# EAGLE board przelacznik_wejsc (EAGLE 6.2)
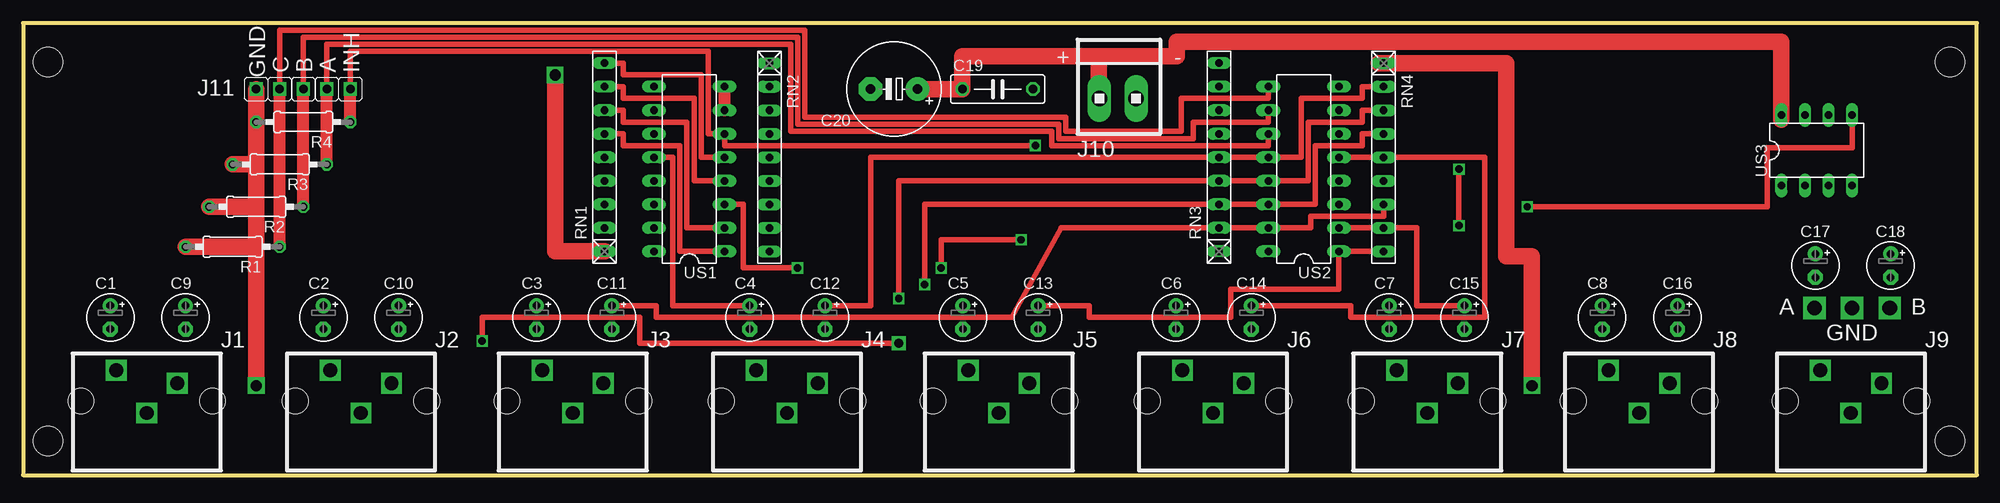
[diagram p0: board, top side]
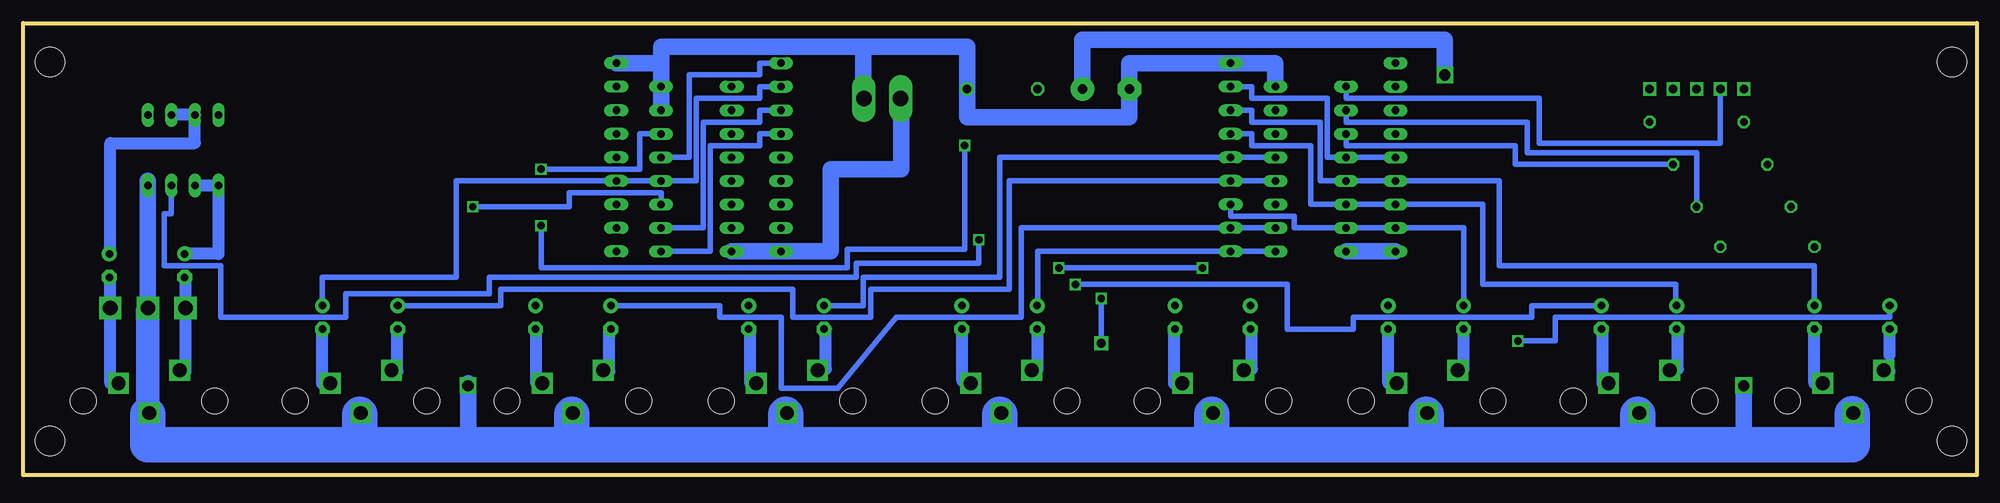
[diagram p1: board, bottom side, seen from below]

Size 210.82 x 48.77 mm. Coordinates in mm from the lower left corner, seen from the top.
Outline: 0,0 210.82,0 210.82,48.77 0,48.77 0,0
Copper layers (1*16): Top 0.035mm / dielectric 1.5mm / Bottom 0.035mm
Design rules: minimum track width 10mil, minimum drill 24mil, track to track 8mil, track to pad 8mil, pad to pad 8mil, via to via 8mil, smd to smd 8mil, copper to edge 40mil, drill to drill 8mil, minimum pad ring 10mil, minimum via ring 8mil, stop-mask expansion 4mil, vias tented up to drill 0mil, thermal gap 10mil
Holes 2.8 mm at 6.23,8 20.43,8 29.35,8 43.55,8 52.21,8 66.41,8 75.32,8 89.52,8 98.18,8 112.38,8 121.3,8 135.5,8 144.41,8 158.61,8 167.27,8 181.47,8 190.13,8 204.33,8
Holes 3.2 mm at 2.68,3.68 207.91,3.68 207.91,44.58 2.68,44.58

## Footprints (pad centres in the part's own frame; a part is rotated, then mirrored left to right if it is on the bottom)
E2,5-5 = drill 0.813 pad 1.6: + -1.27,0 | drill 0.813 pad 1.6 octagon: - 1.27,0
C075-032X103 = drill 0.914 octagon: 1 -3.81,0; 2 3.81,0
E5-10,5 = drill 1.016 pad 2.54: + -2.54,0 | drill 1.016 pad 2.54 octagon: - 2.54,0
JP1 = drill 0.914 pad 1.422 square: 1 0,-1.27; 2 0,1.27
1X2MTA = drill 1.676 long: 1 1.981,0; 2 -1.981,0
0207/10 = drill 0.813 octagon: 1 -5.08,0; 2 5.08,0
RN-9 = drill 0.813 long: 1 -10.16,0; 2 -7.62,0; 3 -5.08,0; 4 -2.54,0; 5 0,0; 6 2.54,0; 7 5.08,0; 8 7.62,0; 9 10.16,0
DIL16 = drill 0.813 long: 1 -8.89,-3.81; 2 -6.35,-3.81; 3 -3.81,-3.81; 4 -1.27,-3.81; 5 1.27,-3.81; 6 3.81,-3.81; 7 6.35,-3.81; 8 8.89,-3.81; 9 8.89,3.81; 10 6.35,3.81; 11 3.81,3.81; 12 1.27,3.81; 13 -1.27,3.81; 14 -3.81,3.81; 15 -6.35,3.81; 16 -8.89,3.81
DIL08 = drill 0.813 long: 1 -3.81,-3.81; 2 -1.27,-3.81; 3 1.27,-3.81; 4 3.81,-3.81; 5 3.81,3.81; 6 1.27,3.81; 7 -1.27,3.81; 8 -3.81,3.81

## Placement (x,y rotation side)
C1  [E2,5-5]  9.4,17.02 270 top
C2  [E2,5-5]  32.4,17.02 270 top
C3  [E2,5-5]  55.4,17.02 270 top
C4  [E2,5-5]  78.4,17.02 270 top
C5  [E2,5-5]  101.4,17.02 270 top
C6  [E2,5-5]  124.4,17.02 270 top
C7  [E2,5-5]  147.4,17.02 270 top
C8  [E2,5-5]  170.4,17.02 270 top
C9  [E2,5-5]  17.53,17.02 270 top
C10  [E2,5-5]  40.53,17.02 270 top
C11  [E2,5-5]  63.53,17.02 270 top
C12  [E2,5-5]  86.53,17.02 270 top
C13  [E2,5-5]  109.53,17.02 270 top
C14  [E2,5-5]  132.53,17.02 270 top
C15  [E2,5-5]  155.53,17.02 270 top
C16  [E2,5-5]  178.53,17.02 270 top
C17  [E2,5-5]  193.4,22.61 270 top
C18  [E2,5-5]  201.53,22.61 270 top
C19  [C075-032X103]  105.16,41.66 0 top
C20  [E5-10,5]  93.98,41.66 180 top
E$9  [JP1]  31.5,41.66 90 top
E$10  [JP1]  28.96,41.66 90 top
E$11  [JP1]  26.42,41.66 90 top
J10  [1X2MTA]  118.11,40.64 0 top
J11  [JP1]  34.04,41.66 90 top
R1  [0207/10]  22.61,24.64 180 top
R2  [0207/10]  25.15,28.96 180 top
R3  [0207/10]  27.69,33.53 180 top
R4  [0207/10]  30.23,38.1 180 top
RN1  [RN-9]  62.74,34.29 90 top
RN2  [RN-9]  80.52,34.29 270 top
RN3  [RN-9]  129.03,34.29 90 top
RN4  [RN-9]  146.81,34.29 270 top
US1  [DIL16]  71.88,33.02 90 top
US2  [DIL16]  138.18,33.02 90 top
US3  [DIL08]  193.55,35.05 0 top

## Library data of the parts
C1-C20 R1-R4 = rcl
E$9-E$11 J11 = hybrid
J10 = con-amp
RN1-RN4 = resistor-net
US1-US3 = 40xx

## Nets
S$9: C9.+ RN2.3 US1.13
S$15: E$11.2 R3.2
S$39: US2.3 US3.5
S$87: RN1.1
S$88: C19.2 C20.- RN2.1 RN4.1 US2.7 US2.8
S$89: C1.+ RN4.3 US2.13
S$90: RN2.4 US1.14
S$91: RN2.7 US1.15
S$92: RN1.5 RN2.2 US1.12
S$93: RN1.6 US1.1
S$94: RN3.1
S$95: RN1.9 US1.5
S$97: RN1.8
S$98: US1.7 US1.8
S$99: US1.4
S$100: US1.2
S$101: RN3.8 US2.4
S$102: RN3.7 US2.2
S$103: RN3.9 US2.5
S$104: RN3.6 RN4.9 US2.1
S$106: RN4.7 US2.15
S$107: US3.4
S$109: US3.6 US3.7
S$111: RN4.2 US2.12
S$113: RN4.4 US2.14
S$116: US1.3 US3.3
S$117: R2.2
S$119: R1.2
S$120: J11.2 R3.1 US1.11 US2.11
S$121: E$9.2 R2.1 US1.10 US2.10
S$123: E$10.2 R1.1 US1.9 US2.9
S$124: R4.1 US1.6 US2.6
S$128: C19.1 C20.+

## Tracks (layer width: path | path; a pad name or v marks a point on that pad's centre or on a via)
S$1  (via drill 1.5)
  other vias: 13.33,6.7
S$2  (via drill 1.5)
  other vias: 16.63,9.9
S$3  (via drill 1.5)
  other vias: 10.03,11.3
S$4  (via drill 1.5)
  other vias: 36.45,6.7
S$5  (via drill 1.5)
  other vias: 39.75,9.9
S$6  (via drill 1.5)
  other vias: 33.15,11.3
S$7
  Bottom 1.27: 33.02,11.43 32.26,11.43 32.26,15.75
S$8
  Bottom 1.27: 39.88,9.91 40.39,9.91 40.39,15.75
S$9
  Bottom 0.61: RN2.3 78.23,39.37 78.23,38.1 70.87,38.1 70.87,31.75 US1.13 51.56,31.75 51.56,22.61 17.53,22.61 C9.+
S$10  (via drill 1.5)
  other vias: 59.31,6.7
S$11  (via drill 1.5)
  other vias: 62.61,9.9
S$12  (via drill 1.5)
  other vias: 56.01,11.3
S$13
  Bottom 1.27: 56.13,11.43 55.37,11.43 55.37,15.75
S$14
  Bottom 1.27: 62.74,9.91 63.5,9.91 63.5,15.75
S$15  (via drill 1.2)
  Top 1.778: 25.15,33.53 E$11.2 | 25.15,33.53 R3.2 | v25.15,9.65 25.15,33.53
  Bottom 1.778: 25.15,5.08 v25.15,9.65
S$16  (via drill 1.5)
  other vias: 82.42,6.7
S$17  (via drill 1.5)
  other vias: 85.72,9.9
S$18  (via drill 1.5)
  other vias: 79.12,11.3
S$19
  Bottom 1.27: 102.11,11.43 101.35,11.43 101.35,15.75
S$20
  Bottom 1.27: 108.46,10.16 109.47,10.16 109.47,15.75
S$21
  Bottom 1.27: 78.99,11.43 78.23,11.43 78.23,15.75
S$22
  Bottom 3.81: 82.55,3.56 82.55,6.56
S$23  (via drill 1.5)
  other vias: 105.28,6.7
S$24  (via drill 1.5)
  other vias: 108.58,9.9
S$25  (via drill 1.5)
  other vias: 101.98,11.3
S$26
  Bottom 1.27: 85.85,9.91 86.61,9.91 86.61,15.75
S$27
  Bottom 1.27: 9.42,12.95 9.42,15.75
S$28  (via drill 1.5)
  other vias: 128.4,6.7
S$29  (via drill 1.5)
  other vias: 131.7,9.9
S$30  (via drill 1.5)
  other vias: 125.1,11.3
S$31
  Bottom 1.27: 124.97,11.43 124.21,11.43 124.21,15.75
S$32
  Bottom 1.27: 131.83,9.91 132.33,9.91 132.33,15.75
S$33  (via drill 1.2)
  Top 1.778: 146.3,44.45 160.02,44.45 160.02,23.62 162.81,23.62 v162.81,9.65
S$34  (via drill 1.5)
  other vias: 151.51,6.7
S$35  (via drill 1.5)
  other vias: 154.81,9.9
S$36  (via drill 1.5)
  other vias: 148.21,11.3
S$37
  Bottom 1.27: 148.34,11.18 147.57,11.18 147.57,15.75
S$38
  Bottom 1.27: 154.94,9.91 155.45,9.91 155.45,15.75
S$39  (via drill 0.8)
  Top 0.61: US3.5 197.36,35.31 188.21,35.31 188.21,28.96 v162.31,28.96
  Bottom 0.61: US2.3 141.99,30.48 151.89,30.48 151.89,28.96 v162.31,28.96
S$40  (via drill 1.5)
  other vias: 174.37,6.7
S$41  (via drill 1.5)
  other vias: 177.67,9.9
S$42  (via drill 1.5)
  other vias: 171.07,11.3
S$43
  Bottom 1.27: 170.43,15.75 170.43,11.18 170.94,11.18
S$45
  Bottom 3.81: 105.41,3.56 105.41,6.56
S$46
  Bottom 3.81: 128.52,3.56 128.52,6.56
S$47
  Bottom 3.81: 151.64,3.56 151.64,6.56
S$48
  Bottom 3.81: 36.58,3.56 36.58,6.56
S$49
  Bottom 3.81: 59.44,3.56 59.44,6.56
S$50
  Bottom 1.27: 177.8,9.91 178.56,9.91 178.56,15.75
S$52
  Bottom 3.81: 174.5,3.56 174.5,6.56
S$53  (via drill 1.5)
  other vias: 197.23,6.7
S$54  (via drill 1.5)
  other vias: 200.53,9.9
S$55  (via drill 1.5)
  other vias: 193.93,11.3
S$56
  Bottom 1.27: 193.29,21.34 193.29,11.18 193.8,11.18
S$57
  Bottom 1.27: 201.42,21.34 201.42,9.91 200.66,9.91
S$59
  Bottom 3.81: 197.36,6.56 197.36,3.3 13.46,3.3 13.46,6.6
S$86
  Bottom 1.27: 16.76,9.91 17.53,9.91 17.53,15.62
S$87
  Top 1.778: RN1.1 57.4,24.13 57.4,43.18
  Bottom 1.27: 68.07,24.13 68.58,24.13
  Bottom 1.778: RN1.1 68.07,24.13
S$88
  Bottom 1.27: 75.69,44.45 RN2.1 91.44,44.45 C20.- 91.44,38.61 | 108.97,38.61 C19.2 108.97,46.23 | 120.14,46.23 120.14,41.66 | 141.99,44.45 141.99,42.16 | US2.8 141.99,39.62 US2.7
  Bottom 1.778: 141.99,44.45 RN4.1 | 141.99,44.45 141.99,39.62 | 141.99,44.45 141.99,46.23 120.14,46.23 | 120.14,46.23 120.14,41.4 | 120.14,46.23 108.97,46.23 108.97,38.61 91.44,38.61 91.44,44.45 75.69,44.45 75.69,42.16
S$89  (via drill 0.8, 1)
  Top 0.61: RN4.3 144.53,39.37 144.53,38.1 138.68,38.1 138.68,31.75 US2.13 94.49,31.75 v94.49,19.05 | v94.49,14.22 66.55,14.22 66.55,17.02 49.53,17.02 v49.53,14.48
  Bottom 0.61: v94.49,14.22 v94.49,19.05 | v49.53,14.48 45.47,14.48 45.47,17.02 9.4,17.02 C1.+ 9.65,18.29
S$90
  Bottom 0.61: RN2.4 78.23,36.83 78.23,35.56 71.88,35.56 71.88,29.21 US1.14 53.34,29.21 53.34,20.57 32.51,20.57 32.51,18.29
S$91
  Bottom 0.61: 55.37,18.29 55.37,26.67 US1.15 73.66,26.67 73.66,27.94 80.52,27.94 RN2.7
S$92
  Top 0.61: US1.12 70.1,34.29 70.1,18.29 78.49,18.29
  Bottom 0.61: RN1.5 US1.12 70.1,34.29 70.1,40.64 78.23,40.64 78.23,41.91 RN2.2
S$93
  Top 0.61: US1.1 70.87,24.13 70.87,35.56 64.77,35.56 64.77,36.83 RN1.6
  Bottom 0.61: US1.1 101.35,24.13 101.35,18.29
S$94
  Bottom 1.27: RN3.1 134.37,24.13 134.87,24.13
  Bottom 1.778: 134.37,24.13 123.7,24.13 123.7,33.02 116.08,33.02 116.08,41.66
S$95
  Top 0.61: US1.5 73.15,34.29 73.15,43.18 64.77,43.18 64.77,44.45 RN1.9
  Bottom 0.61: 124.46,18.29 120.14,18.29 120.14,21.34 105.41,21.34 105.41,34.29 US1.5
S$96
  Bottom 1.27: 9.91,11.18 9.4,11.18
S$97
  Top 0.61: 75.95,31.75 72.39,31.75 72.39,40.64 64.77,40.64 64.77,41.91 RN1.8
S$98
  Top 1.27: US1.7 US1.8
S$99
  Bottom 0.61: 170.43,18.29 159.26,18.29 159.26,20.07 127.76,20.07 127.76,17.02 119.38,17.02 119.38,20.07 104.39,20.07 104.39,31.75 US1.4
S$100
  Top 0.61: US1.2 71.63,26.67 71.63,38.1 64.77,38.1 64.77,39.37 62.74,39.37
  Bottom 0.61: 147.32,18.29 135.64,18.29 135.64,17.02 129.03,17.02 129.03,9.4 122.94,9.4 116.59,17.02 103.12,17.02 103.12,26.67 US1.2
S$101
  Bottom 0.61: 178.56,18.29 178.56,21.34 164.08,21.34 164.08,31.75 US2.4 138.18,31.75 138.18,40.64 131.32,40.64 131.32,41.91 RN3.8
S$102
  Top 0.61: US2.2 150.37,26.67 150.37,18.29 155.45,18.29
  Bottom 0.61: US2.2 137.41,26.67 137.41,38.1 131.32,38.1 131.32,39.37 RN3.7
S$103
  Top 0.61: 132.59,18.29 143.26,18.29 143.26,17.02 157.73,17.02 157.73,34.29 US2.5
  Bottom 0.61: US2.5 138.94,34.29 138.94,43.18 131.32,43.18 131.32,44.45 RN3.9
S$104
  Top 0.61: 109.47,18.29 115.06,18.29 115.06,17.02 130.3,17.02 130.3,20.07 141.99,20.07 US2.1 RN4.9
  Bottom 0.61: US2.1 136.65,24.13 136.65,35.56 131.32,35.56 131.32,36.83 RN3.6
S$105
  Bottom 3.81: 13.46,3.56 13.46,6.56
S$106
  Top 0.61: 63.5,18.29 68.33,18.29 68.33,17.02 106.68,17.02 112.01,26.67 US2.15 138.94,26.67 138.94,27.94 146.81,27.94 RN4.7
S$107  (via drill 1.6)
  Bottom 1.27: US3.4 v197.36,18.03 197.36,17.78
  Bottom 1.778: 197.36,7.11 197.36,17.78 197.36,31.75
  Bottom 2.54: 197.36,6.6 197.36,17.78
S$108
  Bottom 1.27: 189.74,31.24 189.74,31.75 | 189.74,31.24 189.74,23.88 193.29,23.88 | 189.74,31.24 192.02,31.24
S$109
  Bottom 1.27: 201.42,23.88 201.42,35.81 192.28,35.81 US3.7 US3.6
S$111
  Top 0.61: RN4.2 144.53,41.91 144.53,40.64 137.92,40.64 137.92,34.29 US2.12 91.44,34.29 91.44,18.29 86.61,18.29
S$113  (via drill 0.8)
  Top 0.61: RN4.4 144.53,36.83 144.53,35.56 139.45,35.56 139.45,29.21 US2.14 97.28,29.21 v97.28,20.57
  Bottom 0.61: 40.64,18.29 48.01,18.29 48.01,17.02 67.31,17.02 67.31,15.75 74.42,15.75 74.42,20.57 v97.28,20.57
S$114  (via drill 1.6)
  other vias: 193.29,18.03
S$115  (via drill 1.6)
  other vias: 201.42,18.03
S$116  (via drill 0.8)
  Top 0.61: v107.7,25.4 99.06,25.4 v99.06,22.35 | US1.3 77.72,29.21 77.72,22.35 v83.57,22.35
  Bottom 0.61: v107.7,25.4 107.7,22.86 120.9,22.86 120.9,21.34 160.53,21.34 160.53,19.56 176.02,19.56 176.02,17.02 189.48,17.02 189.48,22.61 195.58,22.61 195.58,28.19 194.82,28.19 US3.3 | v83.57,22.35 v99.06,22.35
S$117
  Top 1.778: R2.2 24.89,28.96
S$119
  Top 1.778: R1.2 24.89,24.64
S$120
  Top 0.61: US2.11 134.37,35.56 111,35.56 111,37.08 82.8,37.08 82.8,46.48 32.77,46.48 J11.2
  Top 1.27: R3.1 J11.2
  Bottom 0.61: US1.11 68.07,35.56 49.78,35.56 49.78,33.53 R3.1
S$121
  Top 0.61: US2.10 134.37,38.1 126.24,38.1 126.24,36.32 111.76,36.32 111.76,37.85 83.57,37.85 83.57,47.24 30.23,47.24 E$9.2
  Top 1.27: R2.1 E$9.2
  Bottom 0.61: US1.10 68.07,38.1 48.51,38.1 48.51,34.8 30.23,34.8 R2.1
S$123
  Top 0.61: US2.9 134.37,40.64 124.97,40.64 124.97,37.08 112.52,37.08 112.52,38.61 84.33,38.61 84.33,48.01 27.69,48.01 E$10.2
  Top 1.27: R1.1 E$10.2
  Bottom 0.61: US1.9 68.07,40.64 47.24,40.64 47.24,35.81 27.69,35.81 E$10.2
S$124  (via drill 0.8)
  Top 0.61: v154.94,26.92 v154.94,33.02 | v109.22,35.56 75.69,35.56 US1.6 73.91,36.83 73.91,45.72 35.31,45.72 R4.1
  Top 1.27: R4.1 35.31,41.66
  Bottom 0.61: US2.6 144.27,36.83 144.27,33.02 v154.94,33.02 | v154.94,26.92 154.94,22.35 121.92,22.35 121.92,24.38 109.22,24.38 v109.22,35.56
S$125
  Bottom 1.778: 162.81,3.05 162.81,9.91
S$128  (via drill 1.2)
  Top 1.778: 116.08,45.21 116.08,41.66 | 116.08,45.21 101.35,45.21 C19.1 C20.+ | 116.08,45.21 124.46,45.21 124.46,46.74 189.74,46.74 189.74,38.35
  Bottom 1.778: C20.+ 96.52,46.99 57.4,46.99 v57.4,43.18

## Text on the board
tNames: + | - | GND | C | B | A | INH | J11 | A | B | GND | J1 | J2 | J3 | J4 | J5 | J6 | J7 | J8 | J9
